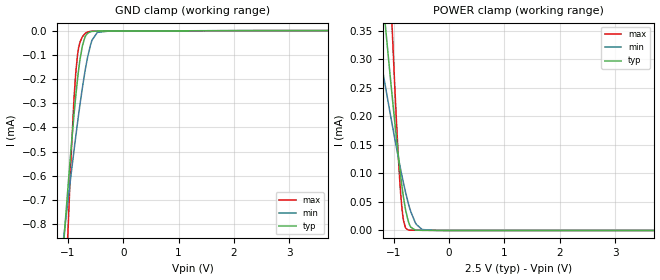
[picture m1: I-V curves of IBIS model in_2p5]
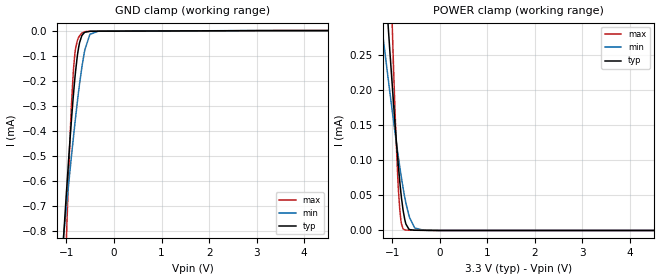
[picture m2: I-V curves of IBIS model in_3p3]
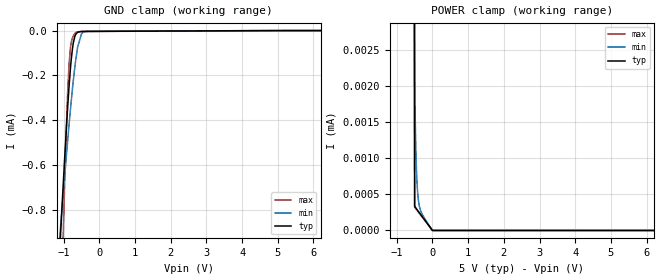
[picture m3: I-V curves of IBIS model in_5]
|Texas Instruments Incorporated
| High-Performance, 5.7kVRMS Reinforced Quad Channel Digital Isolators.
| Marketing part#   Digital Voltage Range   Package-type   #pins
| IS07841DW   2.25V-5.5V   SOIC   16
| IS07841DWR   2.25V-5.5V   SOIC   16
| IS07841DWW   2.25V-5.5V   SOIC   16
| IS07841DWWR   2.25V-5.5V   SOIC   16
[IBIS Ver]   4.1
[File name]   iso7841.ibs
[File Rev]   1.1
[Date]   11/24/2015
[Source]
| Texas Instruments Incorporated.
| Analog-eLab Design Center, HPA
| 12500 TI Blvd
| Dallas, TX -75243
[Notes]   Revision History:
| Rev 1.1: 11/24/2015
| - Add component for package DWW
| Rev 1.0: 12/03/2014
| - Initial version of the model
| - Model generated from simulations in TISPICE
| - Model matched to SPICE simulation
| - C_comp although listed in numerical order of value are
|   obtained from varying PVT conditions. For PVT conditions for
|   each specific value refer the buffer description under
|   respective [Model]. IBIS model user is responsible for using
|   appropriate C_comp to simulate for Signal Integrity.
|* EXCEPTION:   *
|* - For in_* and en_* models there will be leakage current in   *
|*   GROUND clamp because of a resistor(RH2) connected to pad.   *
[Disclaimer]
| This model is designed as an aid for customers of Texas Instruments.
| TI and its licensors and suppliers make no warranties, either expressed
| or implied, with respect to this  model, including the warranties of
| merchantability or fitness for a particular purpose. The model is
| provided solely on an "as is" basis. The entire risk as to its quality
| and performance is with the customer.
[Copyright]
(C) Copyright 2015 Texas Instruments Incorporated.All rights reserved.
|   IS07841DW
[Component]   IS07841DW
[Manufacturer]   TI
[Package]   |16 SOIC - DW package
|   typ   min   max
R_pkg   0.13983   0.12494   0.17928
L_pkg   2.1802nH   1.92454nH   2.85707nH
C_pkg   0.42060pF   0.21450pF   0.61276pF
[Pin]  signal_name   model_name   R_pin   L_pin   C_pin
1   VCC1   POWER   0.09703   2.25823nH  0.63889pF
2   GND1   GND   0.10567   2.15194nH  0.30706pF
3   INA   IN   0.12889   1.99554nH  0.21450pF
4   INB   IN   0.12623   1.94755nH  0.61276pF
5   INC   IN   0.12494   1.92646nH  0.36666pF
6   OUTD   OUT   0.14038   2.18765nH  0.43235pF
7   EN1   EN   0.17807   2.83638nH  0.45904pF
8   GND1   GND   0.08216   2.43955nH  0.44498pF
9   GND2   GND   0.10126   2.44074nH  0.40934pF
10   EN2   EN   0.17928   2.85707nH  0.52717pF
11   IND   IN   0.12883   1.99615nH  0.50841pF
12   OUTC   OUT   0.12617   1.94399nH  0.32633pF
13   OUTB   OUT   0.12498   1.92454nH  0.37783pF
14   OUTA   OUT   0.14050   2.18615nH  0.38097pF
15   GND2   GND   0.08275   2.09014nH  0.75096pF
16   VCC2   POWER   0.09747   2.26909nH  0.67439pF
|   IS07841DWW
[Component]   IS07841DWW
[Manufacturer]   TI
[Package]   |16 SOIC - DWW package
|   typ   min   max
R_pkg   0.2986   0.2007   0.3729
L_pkg   6.1920nH   5.7068nH   6.9814nH
C_pkg   0.3776pF   0.0527pF   0.7658pF
[Pin]  signal_name   model_name   R_pin   L_pin   C_pin
1   VCC1   POWER   0.2515   6.9814nH   0.7658pF
2   GND1   GND   0.2414   6.4743nH   0.4827pF
3   INA   IN   0.3404   6.2419nH   0.3712pF
4   INB   IN   0.2997   5.8575nH   0.3661pF
5   INC   IN   0.3048   5.7068nH   0.3697pF
6   OUTD   OUT   0.3229   5.9972nH   0.3885pF
7   EN1   EN   0.3729   6.6301nH   0.3885pF
8   GND1   GND   0.2162   5.8346nH   0.4827pF
9   GND2   GND   0.2007   6.5823nH   0.5517pF
10   EN2   EN   0.3456   6.8632nH   0.3887pF
11   IND   IN   0.3109   6.1891nH   0.3704pF
12   OUTC   OUT   0.2997   5.7473nH   0.3669pF
13   OUTB   OUT   0.3032   5.8251nH   0.3710pF
14   OUTA   OUT   0.3351   6.1684nH   0.0527pF
15   GND2   GND   0.2007   5.7509nH   0.5517pF
16   VCC2   POWER   0.2768   6.8945nH   0.0527pF
|   Model Selectors
[Model Selector] EN
en_2p5   2.5V digital Input
en_3p3   3.3V digital Input
en_5   5.0V digital Input
[Model Selector] IN
in_2p5   2.5V digital Input
in_3p3   3.3V digital Input
in_5   5.0V digital Input
[Model Selector] OUT
out_2p5   2.5V digital 3-state
out_3p3   3.3V digital 3-state
out_5   5.0V digital 3-state
| Models and submodels in the file (9): in_2p5 (Input), in_3p3 (Input), in_5 (Input), en_2p5 (Input), en_3p3 (Input), en_5 (Input), out_2p5 (3-state), out_3p3 (3-state), out_5 (3-state)
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|   in_2p5 Model
[Model]   in_2p5
Model_type   Input
Vinl = 0.75
Vinh = 1.75
|   typ   min   max
|   (nom PVT)   (fast PVT)   (slow PVT)
C_comp   3.281e-15   3.281e-15   3.250e-14
[Model spec]
|subparameter
Vinl   0.75   0.675   0.825
Vinh   1.75   1.575   1.925
| Where nom  PVT is Nominal Process, 2.5V, 27C
|   Fast PVT is Strong Process,  2.75V, -55C
|   Slow PVT is Weak Process,   2.25V, 150C
[Voltage Range]   2.5   2.25   2.75
|Ambient Temperature   25   125   -55
|Junction Temperature
[Temperature Range]   27   150   -55
[Power Clamp Reference]   2.5   2.25   2.75
[GND Clamp Reference]   0   0   0
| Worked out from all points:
|   GND clamp passes 1 mA (typ) near -1.12 V on its own axis
[GND Clamp]
|   Voltage   I(typ)   I(min)   I(max)
-2.5V     -5.567mA   -3.855mA   -11.2mA
-1.071V   -859.9uA   -843.3uA   -1.249mA
-1.015V   -691.9uA   -732.5uA   -914.2uA
-965mV    -547.7uA   -635.6uA   -635.6uA
-894mV    -356.2uA   -501.7uA   -297uA
-827.5mV  -201.6uA   -381.9uA   -101.5uA
-737.5mV  -61.36uA   -233.7uA   -24.74uA
-643.8mV  -10.62uA   -108.8uA   -5.86uA
-564mV    -3.337uA   -39.15uA   -2.62uA
-468.2mV  -2.078uA   -7.417uA   -2.095uA
-250mV    -1.826uA   -1.892uA   -1.932uA
5V        0A         0A         0A
[POWER Clamp]
|   Voltage   I(typ)   I(min)   I(max)
-2.5V     1.812mA    1.039mA    3.985mA
-1.351V   565.2uA    364.2uA    1.113mA
-1.196V   404.1uA    277.3uA    740.6uA
-1.053V   258.8uA    198.6uA    407.1uA
-990.2mV  197.6uA    165uA      269.2uA
-924.3mV  136.7uA    131uA      139.5uA
-874.8mV  94.88uA    106.6uA    63.72uA
-822.5mV  56.84uA    82.23uA    17.11uA
-740mV    16.82uA    48.51uA    910.2nA
-612.5mV  771.4nA    14.03uA    395.2nA
-486.3mV  326.4nA    1.63uA     313.2nA
5V        0A         0A         0A
|   in_3p3 Model
[Model]   in_3p3
Model_type   Input
Vinl = 0.99
Vinh = 2.31
|   typ   min   max
|   (nom PVT)   (fast PVT)   (slow PVT)
C_comp   3.281e-15   3.281e-15   3.329e-14
[Model spec]
|subparameter
Vinl   0.99   0.891   1.089
Vinh   2.31   2.079   2.541
| Where nom  PVT is Nominal Process, 3.3V, 27C
|   Fast PVT is Strong Process,  3.63V, -55C
|   Slow PVT is Weak Process,   2.97V, 150C
[Voltage Range]   3.3   2.97   3.63
|Ambient Temperature   25   125   -55
|Junction Temperature
[Temperature Range]   27   150   -55
[Power Clamp Reference]   3.3   2.97   3.63
[GND Clamp Reference]   0   0   0
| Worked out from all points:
|   GND clamp passes 1 mA (typ) near -1.12 V on its own axis
|   POWER clamp passes 1 mA (typ) near -1.76 V on its own axis
[GND Clamp]
|   Voltage   I(typ)   I(min)   I(max)
-3.3V     -8.284mA   -5.57mA    -16.97mA
-1.076V   -873.8uA   -852.4uA   -1.277mA
-1.002V   -654.6uA   -707.6uA   -841.1uA
-893.3mV  -354.6uA   -500.5uA   -294.5uA
-853.4mV  -258.1uA   -427.8uA   -159.9uA
-825mV    -196.7uA   -377.6uA   -97.46uA
-772.2mV  -104.4uA   -288.5uA   -41.12uA
-722.7mV  -47.98uA   -211.7uA   -20.38uA
-620.4mV  -7.55uA    -84.56uA   -4.818uA
-505.2mV  -2.819uA   -14.66uA   -2.744uA
-330mV    -2.413uA   -2.673uA   -2.551uA
6.6V      0A         0A         0A
[POWER Clamp]
|   Voltage   I(typ)   I(min)   I(max)
-3.3V     2.693mA    1.517mA    6.009mA
-1.242V   451.1uA    302.7uA    849uA
-1.198V   405.5uA    278.1uA    743.9uA
-1.049V   255uA      196.5uA    398.4uA
-965.9mV  174.7uA    152.3uA    218.9uA
-878.8mV  98.13uA    108.5uA    68.84uA
-842.5mV  70.44uA    91.34uA    30.66uA
-805.2mV  46.22uA    74.6uA     9.403uA
-737.2mV  15.94uA    47.51uA    852.4nA
-526mV    364.9nA    3.505uA    338.9nA
-330mV    219.3nA    268.9nA    212.6nA
6.6V      0A         0A         0A
|   in_5 Model
[Model]   in_5
Model_type   Input
Vinl = 1.5
Vinh = 3.5
|   typ   min   max
|   (nom PVT)   (fast PVT)   (slow PVT)
C_comp   3.281e-15   3.281e-15   3.455e-14
[Model spec]
|subparameter
Vinl   1.5   1.35   1.65
Vinh   3.5   3.15   3.85
| Where nom  PVT is Nominal Process, 5V, 27C
|   Fast PVT is Strong Process,  5.5V, -55C
|   Slow PVT is Weak Process,   4.5V, 150C
[Voltage Range]   5   4.5   5.5
|Ambient Temperature   25   125   -55
|Junction Temperature
[Temperature Range]   27   150   -55
[Power Clamp Reference]   5   4.5   5.5
[GND Clamp Reference]   0   0   0
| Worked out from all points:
|   GND clamp passes 1 mA (typ) near -1.12 V on its own axis
[GND Clamp]
|   Voltage   I(typ)   I(min)   I(max)
-5V       -13.99mA   -9.044mA   -29.25mA
-1.112V   -984.6uA   -924.8uA   -1.503mA
-1.062V   -832.2uA   -825.1uA   -1.194mA
-974mV    -573.5uA   -653.1uA   -684.8uA
-908mV    -392.7uA   -527.9uA   -356.7uA
-850mV    -250.8uA   -421.9uA   -151.8uA
-809mV    -166.1uA   -350.2uA   -74.38uA
-740mV    -65.1uA    -237.9uA   -26.95uA
-608mV    -7.374uA   -73.42uA   -5.426uA
-500mV    -3.903uA   -14.37uA   -3.931uA
-338mV    -3.55uA    -3.864uA   -3.762uA
10V       0A         0A         0A
[POWER Clamp]
|   Voltage   I(typ)   I(min)   I(max)
-5V       185.5mA    66.86mA    305.6mA
-1.007V   213.6uA    173.9uA    305uA
-500mV    338.3nA    2.124uA    322.2nA
-482mV    323.5nA    1.505uA    310.6nA
-473mV    316.7nA    1.273uA    304.8nA
-459.5mV  306.8nA    1.002uA    296.1nA
-432.5mV  288nA      655.7nA    278.7nA
-396.5mV  263.7nA    427.3nA    255.5nA
-360.5mV  239.7nA    320.4nA    232.3nA
-306.5mV  203.8nA    241.2nA    197.5nA
-500uV    0A         0A         0A
10V       0A         0A         0A
